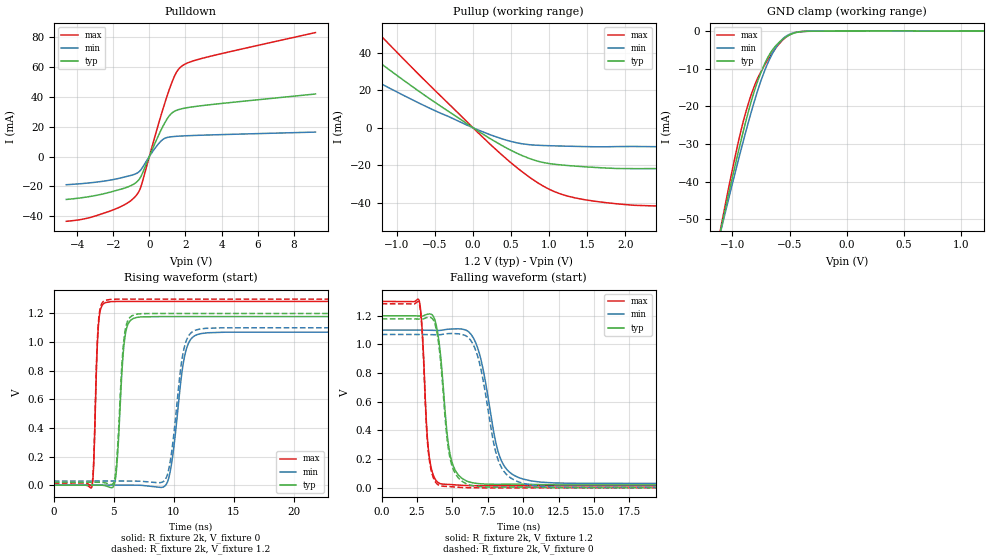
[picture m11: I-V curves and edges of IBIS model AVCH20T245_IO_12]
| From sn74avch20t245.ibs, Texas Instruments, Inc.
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[Model]   AVCH20T245_IO_12
Model_type  I/O
Vinl=0.385
Vinh=0.845
Enable   Active-Low
Vref =   0
Rref =   2000
Cref =   15p
Vmeas =   0.6
| variable   typ   min   max
C_comp   5.41pF   4.73pF   5.93pF
| C_pullup   5.89pF   3.97pF   7.93pF
| C_pulldown   5.44pF   4.83pF   7.13pF
| C_tri-state   5.41pF   4.73pF   5.93pF
[Temperature Range]   40   100   -40
| Ambient temperature   25   85   -40
[Voltage range]   1.2   1.1   1.3
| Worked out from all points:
|   slope of the pulldown table from 0 to 0.18 V, typ, clamps not added: 34.6 ohm
|   slope of the pullup table from 0 to 0.18 V, typ, clamps not added: 38.6 ohm
|   GND clamp passes 1 mA (typ) near -0.50 V on its own axis
|   rising waveform, R_fixture 2k, V_fixture 0: 20-80 % time 474ps typ, 875ps min, 285ps max; typ from 0 V to 1.18 V
|   falling waveform, R_fixture 2k, V_fixture 1.2: 20-80 % time 675ps typ, 1.22ns min, 402ps max; typ from 1.2 V to 0.02 V
|   rising waveform, R_fixture 2k, V_fixture 1.2: 20-80 % time 468ps typ, 857ps min, 283ps max; typ from 0.02 V to 1.2 V
|   falling waveform, R_fixture 2k, V_fixture 0: 20-80 % time 673ps typ, 1.22ns min, 400ps max; typ from 1.18 V to 0 V
[GND Clamp]
| AVCH20T245_IO_12
|   Voltage   I(typ)   I(min)   I(max)
-4.6V     -599.5mA   -548.1mA   -664.5mA
-1.095V   -51.65mA   -52.16mA   -51.03mA
-1.07V    -48.2mA    -49.03mA   -47.15mA
-940mV    -30.92mA   -33.24mA   -28.27mA
-840mV    -19.11mA   -21.95mA   -17.27mA
-775mV    -12.93mA   -15.39mA   -12.23mA
-695mV    -7.282mA   -8.82mA    -7.866mA
-615mV    -3.733mA   -4.168mA   -4.305mA
-545mV    -1.871mA   -1.692mA   -1.969mA
-465mV    -604.4uA   -486.8uA   -527.9uA
-355mV    -86uA      -70.97uA   -92.21uA
1.2V      714.8pA    1.474uA    -44.11nA
[Pulldown]
| AVCH20T245_IO_12
|   Voltage   I(typ)   I(min)   I(max)
-4.6V     -28.79mA   -18.92mA   -43.46mA
-3.415V   -27.06mA   -17.81mA   -41.32mA
-2.035V   -23.45mA   -15.53mA   -35.96mA
-1.17V    -20.3mA    -13.14mA   -30.86mA
-680mV    -16.87mA   -11.13mA   -25.38mA
-435mV    -12.68mA   -8.327mA   -19.06mA
440mV     12.38mA    7.543mA    19.04mA
955mV     24.67mA    12.69mA    39.57mA
1.42V     30.53mA    13.49mA    54.64mA
1.79V     32.04mA    13.78mA    60.61mA
3.17V     34.51mA    14.41mA    66.63mA
9.2V      41.96mA    16.4mA     83.17mA
[Pullup]
| AVCH20T245_IO_12
|   Voltage   I(typ)   I(min)   I(max)
-4.6V     40.24mA    7.956mA    186.3mA
-4.08V    45.4mA     8.808mA    167.8mA
-3.73V    53.62mA    9.647mA    154.2mA
-2.685V   79.31mA    16.98mA    111.4mA
-2.57V    75.87mA    21.96mA    106.5mA
-2.565V   75.72mA    49.42mA    106.3mA
-1.845V   53.66mA    37.03mA    75.82mA
-1.36V    38.76mA    26.71mA    55.3mA
575mV     -13.51mA   -7.977mA   -21.19mA
1.01V     -19.08mA   -9.527mA   -32.92mA
1.455V    -20.71mA   -9.971mA   -38.21mA
9.2V      -28.28mA   -12.48mA   -52.65mA
[Ramp]
| AVCH20T245_IO_12
| variable   typ   min   max
dV/dt_r   0.72/4.87E-10   0.65/8.93E-10   0.78/2.90E-10
dV/dt_f   0.72/6.87E-10   0.65/1.23E-09   0.78/4.15E-10
R_load = 2k
[Rising Waveform]
| AVCH20T245_IO_12
R_fixture =   2k
C_fixture =   0
L_fixture =   0
V_fixture =   0
V_fixture_min = 0
V_fixture_max = 0
|   Time   V(typ)   V(min)   V(max)
0s        18.14nV    102.1nV    431.7pV
3.16ns    600.4uV    -122.3uV   -16.25mV
3.715ns   441.5uV    149.9uV    1.109V
4.31ns    -4.373mV   164.1uV    1.276V
5.125ns   36.02mV    465.4uV    1.284V
5.88ns    1.002V     358.6uV    1.284V
6.695ns   1.167V     197.6uV    1.284V
9.475ns   1.178V     21.29mV    1.284V
11.92ns   1.178V     1.051V     1.284V
40ns      1.178V     1.069V     1.284V
[Falling Waveform]
| AVCH20T245_IO_12
R_fixture =   2k
C_fixture =   0
L_fixture =   0
V_fixture =   1.2
V_fixture_min = 1.1
V_fixture_max = 1.3
|   Time   V(typ)   V(min)   V(max)
0s        1.2V       1.1V       1.3V
2.65ns    1.198V     1.1V       1.304V
3.32ns    1.212V     1.099V     247.9mV
4.13ns    951.3mV    1.098V     29.78mV
4.7ns     313.1mV    1.106V     24.12mV
5.275ns   109.4mV    1.109V     20.25mV
6.775ns   30.34mV    977.7mV    14.82mV
8.445ns   25mV       192.3mV    14.47mV
9.975ns   25.56mV    61.87mV    14.45mV
40ns      20.07mV    28.67mV    14.44mV
[Rising Waveform]
| AVCH20T245_IO_12
R_fixture =   2k
C_fixture =   0
L_fixture =   0
V_fixture =   1.2
V_fixture_min = 1.1
V_fixture_max = 1.3
|   Time   V(typ)   V(min)   V(max)
0s        20.07mV    28.66mV    14.44mV
3.155ns   20.64mV    28.59mV    -1.929mV
3.71ns    20.39mV    28.86mV    1.128V
4.295ns   15.97mV    28.84mV    1.292V
5.1ns     54.55mV    29.04mV    1.3V
5.86ns    1.029V     28.8mV     1.3V
6.66ns    1.189V     28.55mV    1.3V
9.405ns   1.2V       57.09mV    1.3V
11.8ns    1.2V       1.083V     1.3V
40ns      1.2V       1.1V       1.3V
[Falling Waveform]
| AVCH20T245_IO_12
R_fixture =   2k
C_fixture =   0
L_fixture =   0
V_fixture =   0
V_fixture_min = 0
V_fixture_max = 0
|   Time   V(typ)   V(min)   V(max)
0s        1.178V     1.069V     1.284V
2.65ns    1.177V     1.069V     1.287V
3.315ns   1.189V     1.069V     233mV
4.11ns    933.4mV    1.068V     15.42mV
4.675ns   297.5mV    1.076V     9.554mV
5.24ns    93.46mV    1.075V     5.423mV
6.705ns   11.13mV    942.4mV    358.6uV
8.34ns    5.034mV    167mV      26.47uV
9.915ns   5.332mV    33.34mV    7.42uV
40ns      268.9nV    4.463uV    137.7nV
